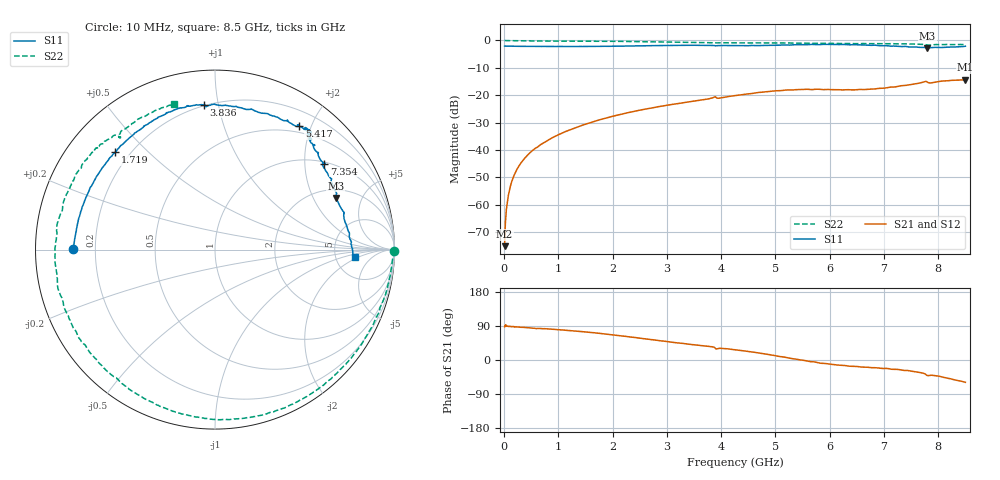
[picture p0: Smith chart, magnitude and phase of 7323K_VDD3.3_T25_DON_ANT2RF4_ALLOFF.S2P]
!Agilent Technologies,E5071C,MY46417908,A.11.23
!Date: Mon Jan 18 17:06:51 2021
!Data & Calibration Information:
!Freq	S11:SOLT2(ON)	S21:SOLT2(ON)	S12:SOLT2(ON)	S22:SOLT2(ON)
!PortZ  Port1:50+j0  Port2:50+j0
!Above PortZ is port z conversion or system Z0 setting when saving the data.
!When reading, reference impedance value at option line is always used.
# Hz S dB R 50
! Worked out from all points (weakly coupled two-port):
!   1601 points, 10 MHz to 8.5 GHz, reference 50 ohm
!   highest |S21| = -14.39 dB at 8.5 GHz (marker M1); lowest = -75.2 dB at 10 MHz (marker M2)
!   lowest |S11| = -2.7 dB at 7.8 GHz (marker M3), VSWR 6.46, Z = 123 + j152 ohm
!   |S11| at or under -10 dB: nowhere
!   |S22| runs from -1.8 to 0.0 dB; largest |S21 - S12| = 0.0035
!   S11 on the Smith chart (normalised r, x): 10 MHz: 0.12, +0.00; 1.719 GHz: 0.15, +0.40; 3.836 GHz: 0.19, +0.91; 5.417 GHz: 0.41, +1.82; 7.354 GHz: 1.05, +2.51; 8.5 GHz: 7.83, -1.75
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1e7  -2.05 179.7  -75.19 87.5  -75.69 87.6  -0.01 -0.4
6.30625e7  -2.08 178.4  -58.52 89.8  -58.55 89.8  -0.07 -2.4
1.055125e8  -2.09 177.3  -54.12 88.7  -54.11 89.1  -0.09 -3.7
1.904125e8  -2.12 175.2  -49.06 87.2  -49.02 87.7  -0.11 -6.4
3.0715e8  -2.16 172.4  -44.91 86.5  -44.88 86.5  -0.13 -10.3
4.822562e8  -2.17 168.2  -40.95 84.7  -40.93 85.0  -0.18 -15.9
7.051188e8  -2.18 162.6  -37.71 82.7  -37.70 82.8  -0.22 -22.8
1.426769e9  -2.20 143.8  -31.10 75.0  -31.11 74.9  -0.30 -44.8
1.718612e9  -2.19 135.6  -29.25 70.9  -29.23 70.9  -0.30 -53.7
2.328831e9  -2.04 120.4  -26.21 60.6  -26.21 60.7  -0.37 -73.7
2.843538e9  -1.91 110.8  -24.22 51.4  -24.23 51.4  -0.50 -92.1
3.835806e9  -1.83 94.3  -21.03 34.9  -21.03 34.9  -0.85 -125.3
4.255e9  -1.89 84.7  -20.17 27.1  -20.18 27.1  -0.88 -136.1
4.8493e9  -1.83 67.6  -18.70 15.0  -18.70 14.8  -0.91 -152.3
5.417069e9  -1.59 55.6  -17.97 1.3  -17.91 1.2  -0.99 -173.8
5.671769e9  -1.44 52.7  -17.99 -4.4  -17.90 -4.4  -1.06 175.2
6.361581e9  -1.59 50.9  -18.02 -16.3  -18.04 -15.8  -1.12 151.0
7.088538e9  -2.01 46.2  -17.13 -22.9  -17.22 -23.0  -1.20 140.5
7.35385e9  -2.22 38.2  -16.49 -27.2  -16.52 -27.1  -1.24 137.9
7.799575e9  -2.71 23.1  -15.22 -41.0  -15.24 -40.9  -1.69 130.3
8.070194e9  -2.57 11.0  -14.83 -44.7  -14.87 -44.7  -1.51 124.2
8.5e9  -2.12 -3.2  -14.39 -58.9  -14.51 -58.9  -1.46 105.8
